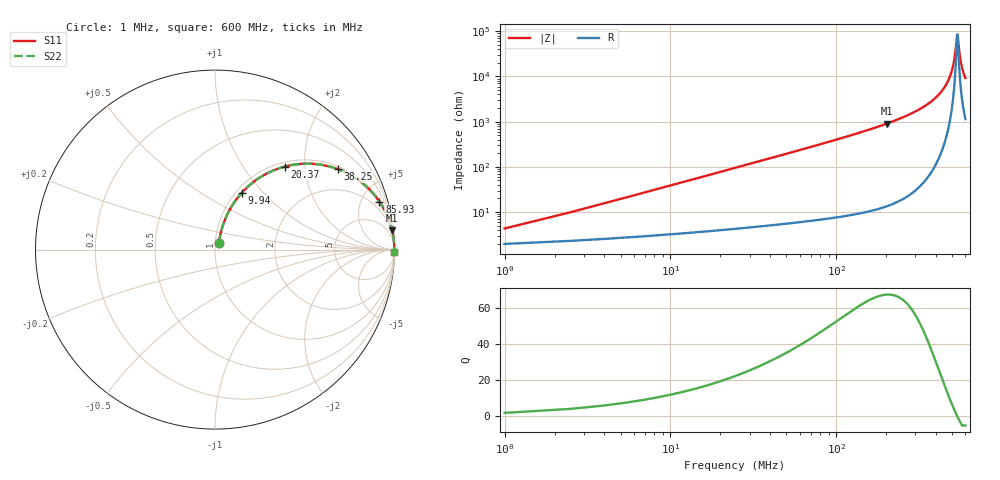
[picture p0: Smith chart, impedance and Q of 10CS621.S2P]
! Coilcraft 1008CS-621 Chip Inductor
! 02 July 2002
# MHZ S MA R 50
!Freq  MagS11  AngS11  MagS21  AngS21  MagS12  AngS12  MagS22  AngS22
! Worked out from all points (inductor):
!   404 points, 1 MHz to 600 MHz, reference 50 ohm
!   read as one part in series: L = 615 nH near 3.98 MHz
!   highest Q = 67.5 at 202.2 MHz (marker M1), where L = 717 nH
!   self-resonance near 535.9 MHz
!   S11 on the Smith chart (normalised r, x): 1 MHz: 1.04, +0.08; 9.94 MHz: 1.06, +0.77; 20.37 MHz: 1.08, +1.58; 38.25 MHz: 1.10, +2.97; 85.93 MHz: 1.14, +6.82; 600 MHz: open
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1  0.04252 60.8  0.9799 -2.2  0.9799 -2.2  0.04252 60.8
5.47  0.2032 71.0  0.9533 -11.6  0.9533 -11.6  0.2032 71.0
9.94  0.3501 64.8  0.908 -20.4  0.908 -20.4  0.3501 64.8
14.41  0.4747 58.0  0.8502 -28.3  0.8502 -28.3  0.4747 58.0
20.37  0.6048 49.9  0.7663 -37.2  0.7663 -37.2  0.6048 49.9
38.25  0.8171 33.3  0.5497 -54.8  0.5497 -54.8  0.8171 33.3
57.62  0.9053 23.7  0.4018 -64.8  0.4018 -64.8  0.9053 23.7
85.93  0.9543 16.3  0.28 -72.6  0.28 -72.6  0.9543 16.3
102.32  0.9674 13.6  0.2357 -75.3  0.2357 -75.3  0.9674 13.6
202.15  0.9924 6.3  0.109 -82.9  0.109 -82.9  0.9924 6.3
301.98  0.9972 3.3  0.05841 -85.6  0.05841 -85.6  0.9972 3.3
401.81  0.9986 1.6  0.02828 -86.4  0.02828 -86.4  0.9986 1.6
462.9  0.9989 0.8  0.01434 -85.1  0.01434 -85.1  0.9989 0.8
501.64  0.9989 0.4  0.00661 -80.1  0.00661 -80.1  0.9989 0.4
516.54  0.9989 0.2  0.003864 -72.9  0.003864 -72.9  0.9989 0.2
532.93  0.9988 0.0  0.001348 -30.7  0.001348 -30.7  0.9988 0.0
537.4  0.9988 -0.0  0.001175 5.7  0.001175 5.7  0.9988 -0.0
540.38  0.9988 -0.0  0.001343 28.8  0.001343 28.8  0.9988 -0.0
552.3  0.9988 -0.2  0.003002 66.2  0.003002 66.2  0.9988 -0.2
562.73  0.9988 -0.3  0.004715 74.6  0.004715 74.6  0.9988 -0.3
579.12  0.9987 -0.4  0.00743 79.7  0.00743 79.7  0.9987 -0.4
600  0.9986 -0.6  0.01083 82.3  0.01083 82.3  0.9986 -0.6
